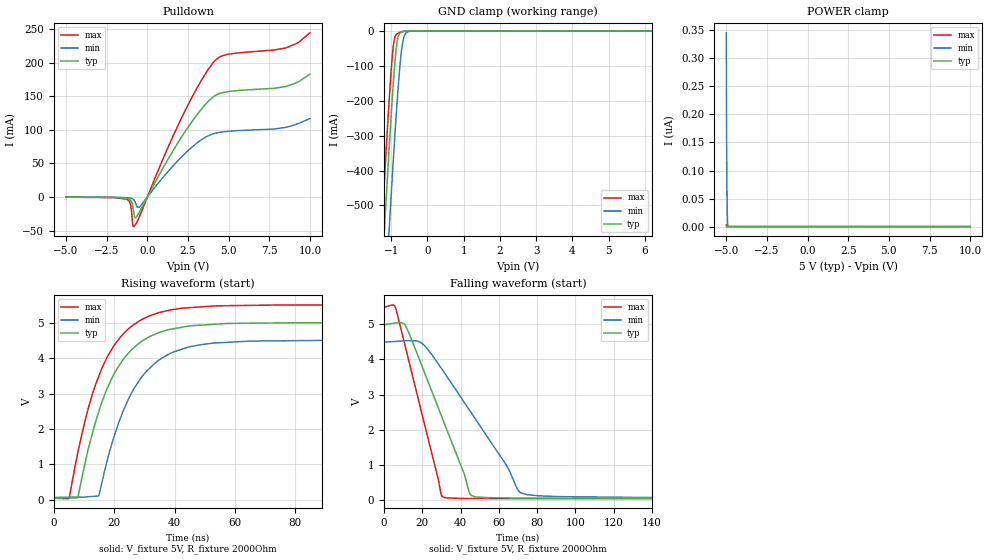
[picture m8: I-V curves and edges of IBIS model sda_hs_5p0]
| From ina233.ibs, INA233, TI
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|   sda_hs_5p0
[Model]   sda_hs_5p0
Model_type   I/O_open_drain
Polarity   Non-Inverting
Vinl = 0.4
Vinh = 3.5
Vmeas = 2.5
Vref = 5.0
Cref = 2pF
Rref = 2000
|   typ   min   max
C_comp   1.140E-12   1.070E-12   1.244E-12
|C_comp_pull_down   1.365E-12   1.341E-12   1.375E-12
| Where Nom  PVT is Nominal Process, 5V, 25C
|   Fast PVT is Strong Process,  5.5V, -40C
|   Slow PVT is Weak Process,   4.5V, 125C
[Voltage Range]   5   4.5   5.5
[Temperature Range]   25   125   -40
[Pullup Reference]   5   4.5   5.5
[Pulldown Reference]   0   0   0
[Power Clamp Reference]   5   4.5   5.5
[GND Clamp Reference]   0   0   0
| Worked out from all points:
|   slope of the pulldown table from 0 to 0.75 V, typ, clamps not added: 22.2 ohm
|   GND clamp passes 1 mA (typ) near -0.66 V on its own axis
|   falling waveform, V_fixture 5V, R_fixture 2000Ohm: 20-80 % time 21.4ns typ, 32.7ns min, 14.9ns max; typ from 5 V to 0.056 V
|   rising waveform, V_fixture 5V, R_fixture 2000Ohm: 20-80 % time 13.1ns typ, 13.3ns min, 12.9ns max; typ from 0.056 V to 5 V
[Pulldown]
|   Voltage   I(typ)   I(min)   I(max)
-5V       -175.5uA   -103.8uA   -209.4uA
-1.25V    -2.156mA   -993.5uA   -3.281mA
-1.04V    -4.675mA   -1.674mA   -10.26mA
-890mV    -14.05mA   -3.009mA   -42.19mA
-830mV    -24.04mA   -4.18mA    -43.88mA
-755mV    -30.86mA   -6.999mA   -42.01mA
-500mV    -22.93mA   -15.27mA   -30.03mA
2.11V     89.43mA    59.83mA    118mA
4.15V     150.6mA    94.7mA     202.6mA
5.05V     157.2mA    97.93mA    212.8mA
8.575V    165mA      104mA      222.5mA
10V       182.9mA    116.8mA    244.4mA
[GND Clamp]
|   Voltage   I(typ)   I(min)   I(max)
-5V       -8.058A    -8.271A    -7.934A
-1.43V    -1.024A    -1.261A    -883mA
-1.25V    -685.5mA   -922.8mA   -543.1mA
-1.16V    -520mA     -756.6mA   -378.3mA
-1.07V    -359.5mA   -593.6mA   -221.2mA
-1.04V    -307.8mA   -540.1mA   -172.1mA
-950mV    -162.4mA   -384.1mA   -50.55mA
-830mV    -27.42mA   -192.9mA   -7.551mA
-710mV    -2.247mA   -51.07mA   -2.53mA
-620mV    -400uA     -9.712mA   -670uA
-410mV    -2.011uA   -80.92uA   -2.42uA
10V       0A         0A         0A
[POWER Clamp]
|   Voltage   I(typ)   I(min)   I(max)
-5V       803.9pA    345.5nA    2.612nA
-4.985V   401.9pA    191.4nA    1.306nA
-4.97V    0A         112.8nA    0A
-4.955V   0A         61.92nA    0A
-4.94V    0A         29.06nA    0A
-4.925V   0A         7.834nA    0A
-4.895V   0A         0A         0A
10V       0A         0A         0A
[Ramp]
R_load = 2000
|   typ   min   max
dV/dt_r   2.96642/1.30968e-08   2.65642/1.33366e-08   3.27147/1.29274e-08
dV/dt_f   2.96642/2.13671e-08   2.65642/3.26847e-08   3.27147/1.49282e-08
[Falling Waveform]
V_fixture = 5V
V_fixture_min = 4.5V
V_fixture_max = 5.5V
R_fixture = 2000Ohm
C_fixture = 0F
|   Time   V(typ)   V(min)   V(max)
0s        5V         4.5V       5.5V
6.131ns   5.034V     4.51V      5.45V
11.68ns   4.912V     4.531V     4.249V
20.25ns   3.754V     4.439V     2.362V
29.82ns   2.423V     3.761V     179.3mV
31.98ns   2.123V     3.588V     73.56mV
45.63ns   143.1mV    2.481V     53.5mV
70.05ns   67.01mV    287.1mV    49mV
75.4ns    65.43mV    155.4mV    48.98mV
500ns     55.96mV    72.64mV    47.54mV
[Rising Waveform]
V_fixture = 5V
V_fixture_min = 4.5V
V_fixture_max = 5.5V
R_fixture = 2000Ohm
C_fixture = 0F
|   Time   V(typ)   V(min)   V(max)
0s        55.96mV    72.64mV    47.54mV
5.091ns   57.17mV    76.69mV    47.86mV
7.997ns   75.59mV    79mV       1.353V
14.86ns   2.487V     119.2mV    3.481V
19.94ns   3.548V     1.783V     4.353V
24.94ns   4.16V      2.883V     4.839V
29.54ns   4.496V     3.513V     5.105V
42ns      4.864V     4.239V     5.403V
88.16ns   4.998V     4.498V     5.498V
500ns     5V         4.5V       5.5V
